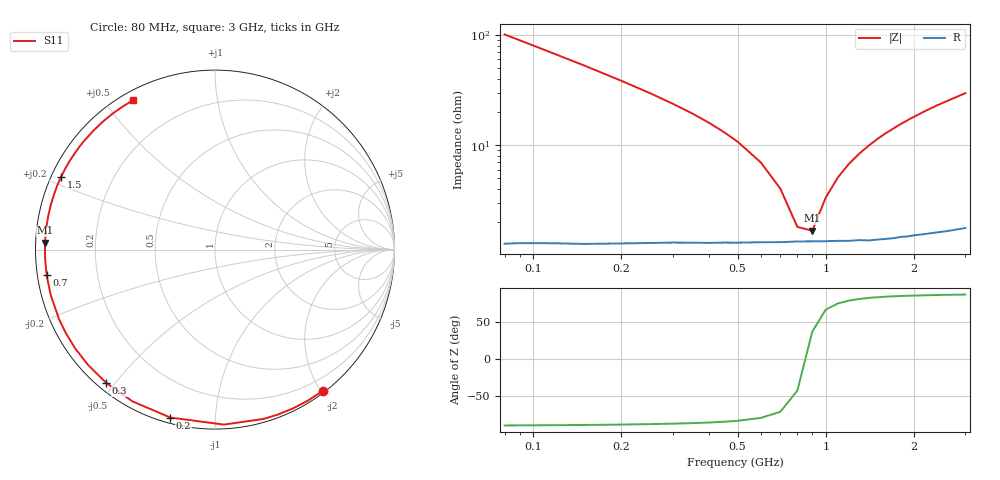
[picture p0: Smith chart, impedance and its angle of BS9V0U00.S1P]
! SIEMENS Small Signal Semiconductors
! BB640
! Si Tuning Diode in SOD323
! VR = 9 V
! S-Parameters:  July  1993
# GHz  S  MA  R  50
!  f  S11
! GHz  MAG  ANG
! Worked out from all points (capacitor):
!   33 points, 80 MHz to 3 GHz, reference 50 ohm
!   read as one part to ground: C = 19.5 pF near 80 MHz
!   lowest |Z| = 1.67 ohm at 900 MHz (marker M1)
!   series resonance near 854.9 MHz, so ESL is about 1.8 nH
!   S11 on the Smith chart (normalised r, x): 80 MHz: 0.03, -2.02; 200 MHz: 0.03, -0.77; 300 MHz: 0.03, -0.47; 700 MHz: 0.03, -0.08; 1.5 GHz: 0.03, +0.23; 3 GHz: 0.04, +0.59
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0.08  0.99 -52.7
0.09  0.9878 -58.4
0.1  0.9857 -63.8
0.11  0.9836 -69.0
0.12  0.9816 -73.9
0.15  0.9762 -87.1
0.2  0.9683 -104.9
0.25  0.9625 -118.5
0.3  0.9583 -129.2
0.35  0.9557 -137.7
0.4  0.954 -144.8
0.45  0.9523 -150.8
0.5  0.9514 -155.9
0.6  0.9497 -164.4
0.7  0.949 -171.3
0.8  0.948 -177.2
0.9  0.9479 177.7
1  0.9479 173.0
1.2  0.9482 164.9
1.3  0.9479 161.3
1.5  0.9485 154.6
1.6  0.9485 151.5
1.8  0.9478 145.7
2  0.9477 140.4
2.2  0.9478 135.4
2.4  0.948 130.8
2.8  0.9486 122.6
3  0.9489 118.8
